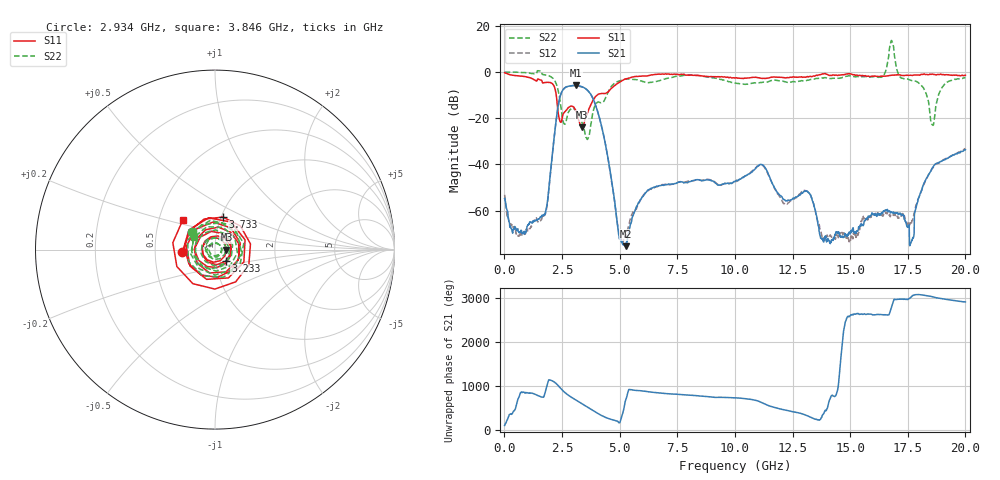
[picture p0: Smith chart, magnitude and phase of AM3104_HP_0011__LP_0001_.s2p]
!Created with skrf (http://scikit-rf.org).
# Hz S RI R 50.0
!freq ReS11 ImS11 ReS21 ImS21 ReS12 ImS12 ReS22 ImS22
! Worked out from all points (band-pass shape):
!   1601 points, 10 MHz to 20 GHz, reference 50 ohm
!   highest |S21| = -5.84 dB at 3.108 GHz (marker M1); lowest = -75.4 dB at 5.257 GHz (marker M2)
!   |S21| within 3 dB of the highest: 2.478 GHz to 3.692 GHz (1.213 GHz wide, 39.3 % of centre)
!   lowest |S11| = -23.9 dB at 3.346 GHz (marker M3), VSWR 1.14, Z = 56.8 - j0.0759 ohm
!   |S11| at or under -10 dB: 2.25 GHz to 4.026 GHz (1.776 GHz wide, 56.6 % of centre)
!   |S22| runs from -29.2 to 13.6 dB; largest |S21 - S12| = 0.028
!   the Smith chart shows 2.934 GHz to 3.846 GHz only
!   S11 on the Smith chart (normalised r, x): 2.934 GHz: 0.69, -0.02; 3.233 GHz: 1.11, -0.15; 3.733 GHz: 1.02, +0.38; 3.846 GHz: 0.66, +0.23
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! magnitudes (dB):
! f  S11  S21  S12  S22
! 10 MHz  -0.3  -54.8  -53.2  0.0
! 597.2 MHz  -1.7  -68.7  -70.8  -0.1
! 1.697 GHz  -4.7  -62.1  -62.2  -1.1
! 2.384 GHz  -20.4  -12.0  -12.0  -10.6
! 2.934 GHz  -14.8  -5.9  -6.0  -15.7
! 3.108 GHz  -17.0  -5.8  -5.8  -17.0
! 3.233 GHz  -21.1  -6.0  -6.1  -18.7
! 3.346 GHz  -23.9  -6.3  -6.4  -20.9
! 3.733 GHz  -14.6  -9.4  -9.4  -23.8
! 3.846 GHz  -12.3  -11.5  -11.5  -17.2
! 4.983 GHz  -4.5  -71.6  -71.2  -3.9
! 5.257 GHz  -3.0  -75.4  -71.2  -3.0
! 6.682 GHz  -0.9  -49.3  -49.4  -3.9
! 10.01 GHz  -2.6  -47.5  -47.7  -4.8
! 11.15 GHz  -2.8  -40.0  -40.2  -4.6
! 12.14 GHz  -2.5  -55.3  -56.9  -4.1
! 13.34 GHz  -2.0  -55.0  -54.8  -3.3
! 14.08 GHz  -1.4  -73.0  -71.0  -2.9
! 16.68 GHz  -1.6  -60.4  -61.9  7.2
! 17.68 GHz  -1.5  -72.8  -64.5  -3.8
! 18.58 GHz  -0.9  -41.3  -41.7  -23.0
! 20 GHz  -1.4  -33.6  -33.2  -2.5
